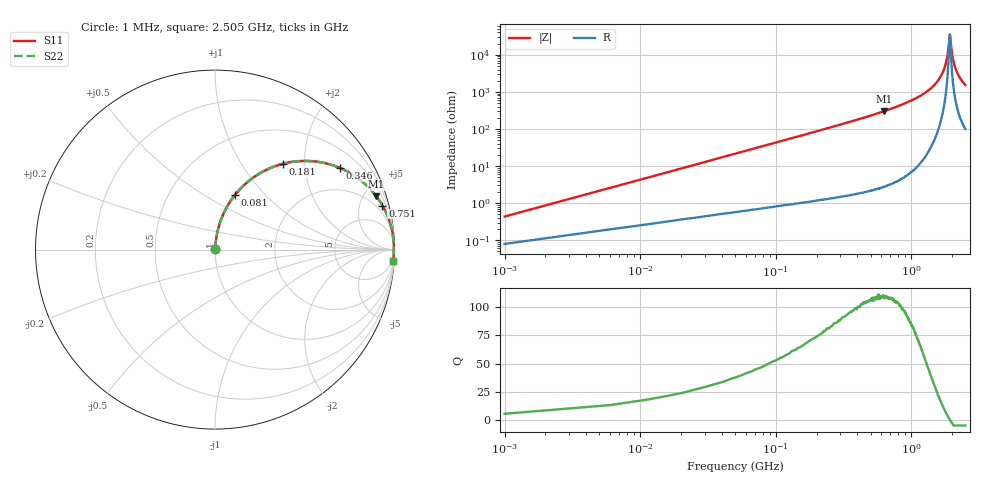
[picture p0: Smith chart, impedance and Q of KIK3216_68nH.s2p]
!version-2
!date-01.2022
!Series
# MHz S RI R 50
!Freq ReS11 ImS11 ReS21 ImS21 ReS12 ImS12 ReS22 ImS22
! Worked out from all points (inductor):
!   501 points, 1 MHz to 2.505 GHz, reference 50 ohm
!   read as one part in series: L = 68 nH near 11 MHz
!   highest Q = 110 at 631 MHz (marker M1), where L = 76.2 nH
!   self-resonance near 1.92 GHz
!   S11 on the Smith chart (normalised r, x): 1 MHz: 1.00, +0.01; 81 MHz: 1.01, +0.69; 181 MHz: 1.02, +1.56; 346 MHz: 1.03, +3.06; 751 MHz: 1.07, +7.58; 2.505 GHz: 3, -31
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1  0.000821 0.00427  0.9992 -0.00427  0.9992 -0.00427  0.000821 0.00427
16  0.00781 0.0676  0.9922 -0.0676  0.9922 -0.0676  0.00781 0.0676
26  0.0161 0.1089  0.9839 -0.1089  0.9839 -0.1089  0.0161 0.1089
46  0.0421 0.1874  0.9579 -0.1874  0.9579 -0.1874  0.0421 0.1874
81  0.1124 0.3055  0.8876 -0.3055  0.8876 -0.3055  0.1124 0.3055
181  0.3801 0.4784  0.6199 -0.4784  0.6199 -0.4784  0.3801 0.4784
346  0.6982 0.4538  0.3018 -0.4538  0.3018 -0.4538  0.6982 0.4538
421  0.7789 0.4101  0.2211 -0.4101  0.2211 -0.4101  0.7789 0.4101
631  0.8991 0.2966  0.1009 -0.2966  0.1009 -0.2966  0.8991 0.2966
751  0.9328 0.2456  0.0672 -0.2456  0.0672 -0.2456  0.9328 0.2456
836  0.9491 0.2149  0.0509 -0.2149  0.0509 -0.2149  0.9491 0.2149
1255  0.9866 0.1061  0.0134 -0.1061  0.0134 -0.1061  0.9866 0.1061
1500  0.9941 0.061  0.0059 -0.061  0.0059 -0.061  0.9941 0.061
1675  0.9965 0.0338  0.00353 -0.0338  0.00353 -0.0338  0.9965 0.0338
1825  0.9972 0.0129  0.0028 -0.0129  0.0028 -0.0129  0.9972 0.0129
1865  0.9972 0.00766  0.00277 -0.00766  0.00277 -0.00766  0.9972 0.00766
1910  0.9972 0.00187  0.0028 -0.00187  0.0028 -0.00187  0.9972 0.00187
1925  0.9972 -2.71e-05  0.00282 2.71e-05  0.00282 2.71e-05  0.9972 -2.71e-05
2000  0.9969 -0.0093  0.00306 0.0093  0.00306 0.0093  0.9969 -0.0093
2090  0.9964 -0.02  0.00357 0.02  0.00357 0.02  0.9964 -0.02
2255  0.9949 -0.0385  0.00505 0.0385  0.00505 0.0385  0.9949 -0.0385
2505  0.9916 -0.0641  0.00839 0.0641  0.00839 0.0641  0.9916 -0.0641
